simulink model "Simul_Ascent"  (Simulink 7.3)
settings: Solver=ode45  StartTime=0.0  StopTime=20  FixedStep=0.0005  MaxStep=0.015  RelTol=1e-3
InitFcn:
  | init
StartFcn:
  | init
StopFcn:
  | pl
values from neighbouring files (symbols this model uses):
  Ave = [    [vehicle_sim.m]
  Bve = [    [vehicle_sim.m]
  Cve = [    [vehicle_sim.m]
  d2r = pi/180    (= 0.0174532925199)    [init.m]    (also in robust.m)
  Dve = [    [vehicle_sim.m]
  r2d = 180/pi    (= 57.2957795131)    [init.m]    (also in robust.m)
undefined symbols (not defined in the file or in its folder): Kmix, Kpr, Kq

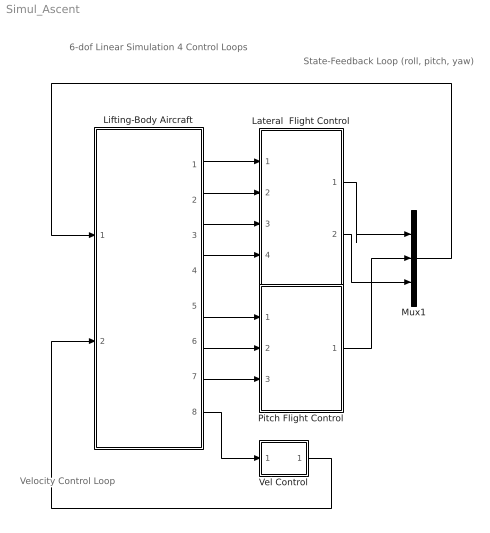
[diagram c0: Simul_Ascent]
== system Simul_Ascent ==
  note: 6-dof Linear Simulation 4 Control Loops
  note: State-Feedback Loop (roll, pitch, yaw)
  note: Velocity Control Loop
  Lateral  Flight Control : Subsystem
  Lifting-Body Aircraft : Subsystem
  Mux1 : Mux  Inputs=3
  Pitch Flight Control : Subsystem
  Vel Control : Subsystem
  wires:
  Lifting-Body Aircraft/6(q) -> Pitch Flight Control/2(q)
  Lifting-Body Aircraft/7(Nz) -> Pitch Flight Control/3(Nz)
  Lifting-Body Aircraft/5(thet) -> Pitch Flight Control/1(theta)
  Lifting-Body Aircraft/4(Ny) -> Lateral  Flight Control/4(Ny)
  Mux1/1 -> Lifting-Body Aircraft/1(PQR dem)
  Pitch Flight Control/1(dQ) -> Mux1/2
  Lifting-Body Aircraft/1(phi) -> Lateral  Flight Control/1(phi)
  Lifting-Body Aircraft/2(p) -> Lateral  Flight Control/2(pb)
  Lifting-Body Aircraft/3(r) -> Lateral  Flight Control/3(rb)
  Lateral  Flight Control/1(dP) -> Mux1/1
  Lateral  Flight Control/2(dR) -> Mux1/3
  Lifting-Body Aircraft/8(Vd) -> Vel Control/1(Vdot)
  Vel Control/1(Ax) -> Lifting-Body Aircraft/2(Ax)

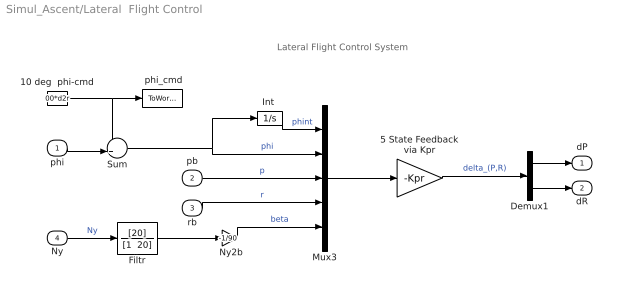
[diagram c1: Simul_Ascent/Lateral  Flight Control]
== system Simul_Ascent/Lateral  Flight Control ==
  note: Lateral Flight Control System
  phi : Inport  OutDataType=sfix(16)  OutScaling=2^0
  pb : Inport  Port=2  OutDataType=sfix(16)  OutScaling=2^0
  rb : Inport  Port=3  OutDataType=sfix(16)  OutScaling=2^0
  Ny : Inport  Port=4  OutDataType=sfix(16)  OutScaling=2^0
  " Ny2b" : Gain  Gain=-1/90  ParameterDataType=sfix(16)  ParameterScaling=2^0  OutDataType=sfix(16)  OutScaling=2^0
  " phi_cmd" : ToWorkspace  VariableName=phicmd  SampleTime=-1  SaveFormat=Array
  10 deg  phi-cmd : Constant  Value=00*d2r  OutDataType=sfix(16)  OutScaling=2^0
  5 State Feedback via Kpr : Gain  Gain=-Kpr  Multiplication=Matrix(K*u)  ParameterDataType=sfix(16)  ParameterScaling=2^0  OutDataType=sfix(16)  OutScaling=2^0
  Demux1 : Demux  Outputs=2
  Filtr : TransferFcn  Numerator=[20]  Denominator="[1  20]"
  "Int " : Integrator
  Mux3 : Mux  Inputs=5
  Sum : Sum  Inputs=-+|  OutDataType=sfix(16)  OutScaling=2^0
  dP : Outport  OutDataType=sfix(16)  OutScaling=2^0
  dR : Outport  Port=2  OutDataType=sfix(16)  OutScaling=2^0
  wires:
  10 deg  phi-cmd/1 -> " phi_cmd"/1, Sum/1
  rb/1 -> Mux3/4  "r"
  pb/1 -> Mux3/3  "p"
  Ny/1 -> Filtr/1  "Ny"
  5 State Feedback via Kpr/1 -> Demux1/1  "delta_(P,R)"
  Demux1/1 -> dP/1
  Demux1/2 -> dR/1
  Sum/1 -> Mux3/2, "Int "/1  "phi"
  "Int "/1 -> Mux3/1  "phint"
  phi/1 -> Sum/2
  Mux3/1 -> 5 State Feedback via Kpr/1
  " Ny2b"/1 -> Mux3/5  "beta"
  Filtr/1 -> " Ny2b"/1

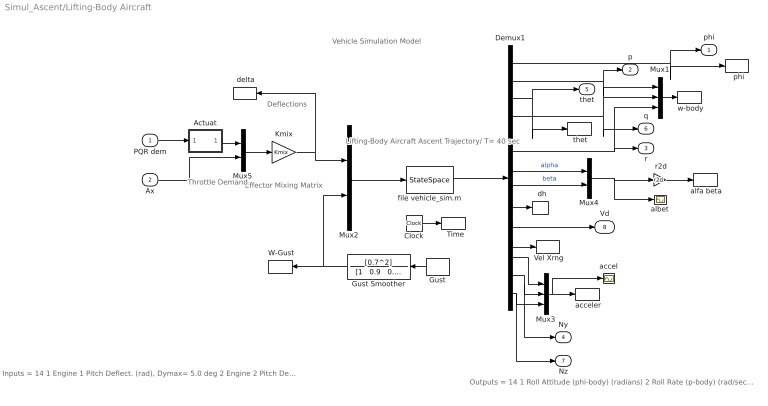
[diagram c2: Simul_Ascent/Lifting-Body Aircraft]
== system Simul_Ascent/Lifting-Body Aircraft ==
  note: Deflections
  note: Vehicle Simulation Model
  note: Outputs = 14 1 Roll Attitude (phi-body) (radians) 2 Roll Rate (p-body) (rad/sec) 3 Pitch Attitude (thet-bdy) (radians) 4 Pitch Rate (q-body) (rad/sec) 5 Yaw Attitude (psi-body) (radians) 6 Yaw Rate (r-body) (rad/sec) 7 Angle of attack, alfa, (radians) 8 Angle of sideslip, beta, (radian) 9 Change in Altitude, delta-h, (feet) 10 Forward Acceleration (V-dot) (ft/sec) 11 Cross Range Velocity (Vcr) (ft/sec) 12 CG Acceleration along X axis, (ft/sec^2) 13 CG Acceleration along Y axis, (ft/sec^2) 14 CG Acceleration along Z axis, (ft/sec^2)
  note: Effector Mixing Matrix
  note: Lifting-Body Aircraft Ascent Trajectory/ T= 40 sec
  note: Inputs = 14 1 Engine 1 Pitch Deflect. (rad), Dymax= 5.0 deg 2 Engine 2 Pitch Deflect. (rad), Dymax= 5.0 deg 3 Engine 1 Yaw Deflection (rad), Dzmax= 5.0 deg 4 Engine 2 Yaw Deflection (rad), Dzmax= 5.0 deg 5 Throttle Input dTh/Th for Engine No1 (-) 6 Throttle Input dTh/Th for Engine No2 (-) 7 LeftElevon Deflection (radians) 8 Right Elevon Deflection (radians) 9 Vertical Rudder Deflection (radians) 10 Upper-Left Body-Flap Deflection(radians) 11 Upper-Right Body-Flap Deflection (radians) 12 Lower-Left Body-Flap Deflection(radians) 13 Lower-Right Body-Flap Deflection (radians) 14 Wind Gust Azim, Elev Angles=(45,90) (deg)
  note: Throttle Demand
  PQR dem : Inport  OutDataType=sfix(16)  OutScaling=2^0
  Ax : Inport  Port=2  OutDataType=sfix(16)  OutScaling=2^0
  "  Time" : ToWorkspace  VariableName=time  SampleTime=-1  SaveFormat=Array
  "  dh" : ToWorkspace  VariableName=dh  SampleTime=-1  SaveFormat=Array
  "  phi" : ToWorkspace  VariableName=phi  SampleTime=-1  SaveFormat=Array
  " Vel Xrng" : ToWorkspace  VariableName=VXR  SampleTime=-1  SaveFormat=Array
  " W-Gust" : ToWorkspace  VariableName=gust  SampleTime=-1  SaveFormat=Array
  " acceler" : ToWorkspace  VariableName=accel  SampleTime=-1  SaveFormat=Array
  " alfa beta" : ToWorkspace  VariableName=albet  SampleTime=-1  SaveFormat=Array
  " delta" : ToWorkspace  VariableName=delta  SampleTime=-1  SaveFormat=Array
  " r2d" : Gain  Gain=r2d  ParameterDataType=sfix(16)  ParameterScaling=2^0  OutDataType=sfix(16)  OutScaling=2^0
  " thet" : ToWorkspace  VariableName=theta  SampleTime=-1  SaveFormat=Array
  " w-body" : ToWorkspace  VariableName=pqr  SampleTime=-1  SaveFormat=Array
  Actuat : Subsystem
  Clock : Clock
  Demux1 : Demux  Outputs=14
  Gust : DiscretePulseGenerator  PulseType=Time based  Amplitude=00  Period=300  PulseWidth=2  PhaseDelay=30  SampleTime=1
  Gust Smoother : TransferFcn  Numerator=[0.7^2]  Denominator="[1   0.9   0.7^2]"
  Kmix : Gain  Gain=Kmix  Multiplication=Matrix(K*u)  ParameterDataType=sfix(16)  ParameterScaling=2^0  OutDataType=sfix(16)  OutScaling=2^0
  Mux1 : Mux  Inputs=3
  Mux2 : Mux  Inputs=[13, 1]
  Mux3 : Mux  Inputs=3
  Mux4 : Mux  Inputs=2
  Mux5 : Mux  Inputs=[3, 1]
  accel : Scope
  albet : Scope
  file vehicle_sim.m : StateSpace  A=Ave  B=Bve  C=Cve  D=Dve
  phi : Outport  OutDataType=sfix(16)  OutScaling=2^0
  p : Outport  Port=2  OutDataType=sfix(16)  OutScaling=2^0
  r : Outport  Port=3  OutDataType=sfix(16)  OutScaling=2^0
  Ny : Outport  Port=4  OutDataType=sfix(16)  OutScaling=2^0
  thet : Outport  Port=5  OutDataType=sfix(16)  OutScaling=2^0
  q : Outport  Port=6  OutDataType=sfix(16)  OutScaling=2^0
  Nz : Outport  Port=7  OutDataType=sfix(16)  OutScaling=2^0
  Vd : Outport  Port=8  OutDataType=sfix(16)  OutScaling=2^0
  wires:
  Mux2/1 -> file vehicle_sim.m/1
  Kmix/1 -> Mux2/1, " delta"/1
  Demux1/2 -> Mux1/1, p/1
  Demux1/4 -> Mux1/2, q/1
  Demux1/6 -> r/1, Mux1/3
  Demux1/7 -> Mux4/1  "alpha"
  Demux1/8 -> Mux4/2  "beta"
  PQR dem/1 -> Actuat/1(in)
  Demux1/1 -> phi/1, "  phi"/1
  file vehicle_sim.m/1 -> Demux1/1
  Demux1/9 -> "  dh"/1
  Demux1/10 -> Vd/1
  Demux1/11 -> " Vel Xrng"/1
  Gust/1 -> Gust Smoother/1
  Gust Smoother/1 -> " W-Gust"/1, Mux2/2
  Mux1/1 -> " w-body"/1
  Demux1/12 -> Mux3/1
  Demux1/14 -> Mux3/3, Nz/1
  Mux3/1 -> " acceler"/1, accel/1
  Clock/1 -> "  Time"/1
  " r2d"/1 -> " alfa beta"/1
  Mux4/1 -> " r2d"/1, albet/1
  Demux1/3 -> thet/1, " thet"/1
  Actuat/1(ou) -> Mux5/1
  Ax/1 -> Mux5/2
  Mux5/1 -> Kmix/1
  Demux1/13 -> Ny/1, Mux3/2

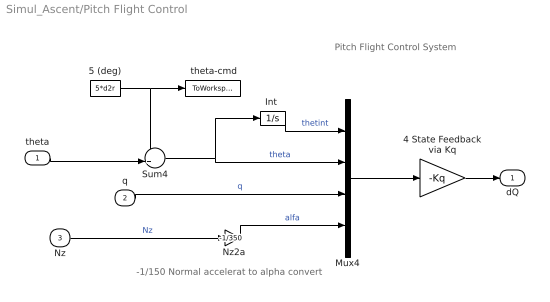
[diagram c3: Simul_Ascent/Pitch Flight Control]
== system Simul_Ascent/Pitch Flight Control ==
  note: Pitch Flight Control System
  note: -1/150 Normal accelerat to alpha convert
  theta : Inport  OutDataType=sfix(16)  OutScaling=2^0
  q : Inport  Port=2  OutDataType=sfix(16)  OutScaling=2^0
  Nz : Inport  Port=3  OutDataType=sfix(16)  OutScaling=2^0
  " Nz2a" : Gain  Gain=-1/350  ParameterDataType=sfix(16)  ParameterScaling=2^0  OutDataType=sfix(16)  OutScaling=2^0
  " theta-cmd" : ToWorkspace  VariableName=Thecmd  SampleTime=-1  SaveFormat=Array
  4 State Feedback via Kq : Gain  Gain=-Kq  Multiplication=Matrix(K*u)  ParameterDataType=sfix(16)  ParameterScaling=2^0  OutDataType=sfix(16)  OutScaling=2^0
  5 (deg) : Constant  Value=5*d2r  OutDataType=sfix(16)  OutScaling=2^0
  "Int " : Integrator
  Mux4 : Mux
  Sum4 : Sum  Inputs=-+|  OutDataType=sfix(16)  OutScaling=2^0
  dQ : Outport  OutDataType=sfix(16)  OutScaling=2^0
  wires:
  q/1 -> Mux4/3  "q"
  Sum4/1 -> Mux4/2, "Int "/1  "theta"
  5 (deg)/1 -> " theta-cmd"/1, Sum4/1
  " Nz2a"/1 -> Mux4/4  "alfa"
  Nz/1 -> " Nz2a"/1  "Nz"
  4 State Feedback via Kq/1 -> dQ/1
  "Int "/1 -> Mux4/1  "thetint"
  theta/1 -> Sum4/2
  Mux4/1 -> 4 State Feedback via Kq/1

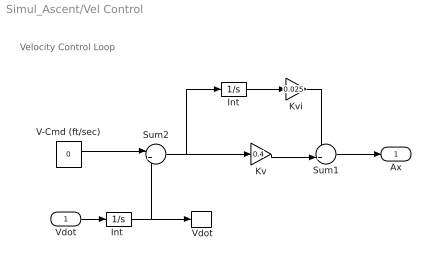
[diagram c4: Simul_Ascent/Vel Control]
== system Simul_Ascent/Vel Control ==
  note: Velocity Control Loop
  Vdot : Inport
  " Vdot" : ToWorkspace  VariableName=dV  SampleTime=-1  SaveFormat=Array
  Int : Integrator
  "Int " : Integrator
  Kv : Gain  Gain=0.4  ParameterDataType=fixdt(1, 16)  ParameterScaling=2^0  OutDataType=fixdt(1, 16)  OutScaling=2^0
  Kvi : Gain  Gain=0.025  ParameterDataType=fixdt(1, 16)  ParameterScaling=2^0  OutDataType=fixdt(1, 16)  OutScaling=2^0
  Sum1 : Sum  Inputs=++|  OutDataType=fixdt(1, 16)  OutScaling=2^0
  Sum2 : Sum  Inputs=|+-  OutDataType=fixdt(1, 16)  OutScaling=2^0
  V-Cmd (ft/sec) : Constant  Value=0  OutDataType=fixdt(1, 16)  OutScaling=2^0
  Ax : Outport
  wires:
  V-Cmd (ft/sec)/1 -> Sum2/1
  Sum2/1 -> Kv/1, Int/1
  Int/1 -> Kvi/1
  Kv/1 -> Sum1/2
  Kvi/1 -> Sum1/1
  Sum1/1 -> Ax/1
  Vdot/1 -> "Int "/1
  "Int "/1 -> Sum2/2, " Vdot"/1

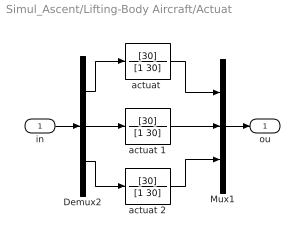
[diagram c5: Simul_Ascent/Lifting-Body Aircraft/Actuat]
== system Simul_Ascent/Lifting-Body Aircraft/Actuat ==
  in : Inport
  Demux2 : Demux  Outputs=3
  Mux1 : Mux  Inputs=3
  "actuat " : TransferFcn  Numerator=[30]  Denominator=[1 30]
  actuat 1 : TransferFcn  Numerator=[30]  Denominator=[1 30]
  actuat 2 : TransferFcn  Numerator=[30]  Denominator=[1 30]
  ou : Outport
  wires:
  actuat 1/1 -> Mux1/2
  "actuat "/1 -> Mux1/1
  actuat 2/1 -> Mux1/3
  Demux2/2 -> actuat 1/1
  Demux2/1 -> "actuat "/1
  Demux2/3 -> actuat 2/1
  in/1 -> Demux2/1
  Mux1/1 -> ou/1
